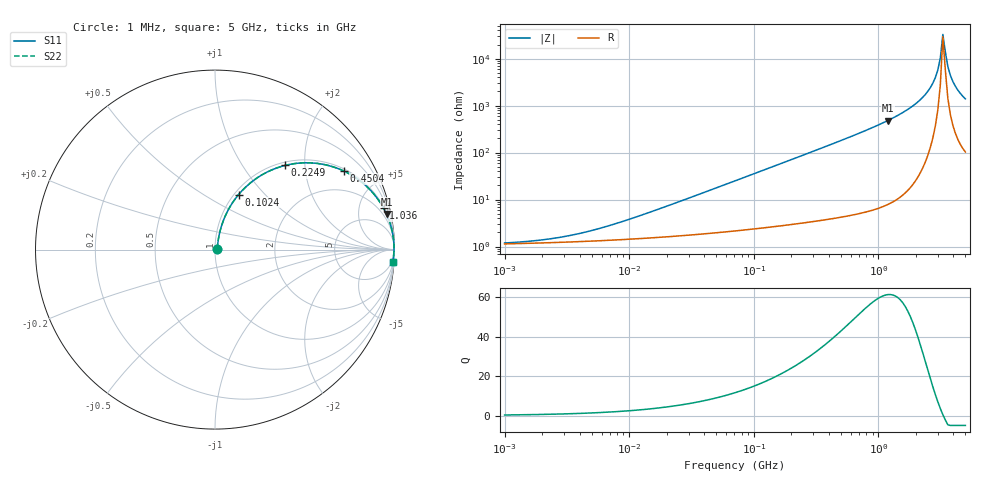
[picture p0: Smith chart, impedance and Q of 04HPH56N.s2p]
# MHz S MA R 50
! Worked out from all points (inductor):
!   185 points, 1 MHz to 5 GHz, reference 50 ohm
!   read as one part in series: L = 56 nH near 12.75 MHz
!   highest Q = 61.4 at 1.191 GHz (marker M1), where L = 64.3 nH
!   self-resonance near 3.296 GHz
!   S11 on the Smith chart (normalised r, x): 1 MHz: 1.02, +0.01; 102.4 MHz: 1.05, +0.72; 224.9 MHz: 1.06, +1.59; 450.4 MHz: 1.08, +3.23; 1.036 GHz: 1.13, +8.08; 5 GHz: 3, -28
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1  0.01176 17.0  0.9888 -0.2  0.9888 -0.2  0.01176 17.0
2.19661  0.01412 32.3  0.9881 -0.4  0.9881 -0.4  0.01412 32.3
4.19948  0.01929 48.3  0.9873 -0.8  0.9873 -0.8  0.01929 48.3
17.6357  0.06291 72.3  0.9827 -3.5  0.9827 -3.5  0.06291 72.3
70.7107  0.2376 71.4  0.9512 -13.7  0.9512 -13.7  0.2376 71.4
102.402  0.333 66.8  0.9213 -19.4  0.9213 -19.4  0.333 66.8
224.938  0.6113 50.1  0.7683 -37.7  0.7683 -37.7  0.6113 50.1
296.948  0.714 42.6  0.6776 -45.5  0.6776 -45.5  0.714 42.6
450.411  0.8409 31.4  0.5207 -57.2  0.5207 -57.2  0.8409 31.4
1036.25  0.967 13.8  0.2394 -75.2  0.2394 -75.2  0.967 13.8
1190.62  0.9759 11.7  0.203 -77.4  0.203 -77.4  0.9759 11.7
1247.03  0.9784 11.0  0.1915 -78.0  0.1915 -78.0  0.9784 11.0
1981.11  0.9937 5.3  0.09186 -83.4  0.09186 -83.4  0.9937 5.3
2615.33  0.997 2.4  0.04125 -84.6  0.04125 -84.6  0.997 2.4
2869.02  0.9973 1.4  0.02522 -83.2  0.02522 -83.2  0.9973 1.4
3004.94  0.9974 1.0  0.01734 -80.9  0.01734 -80.9  0.9974 1.0
3147.31  0.9974 0.5  0.009597 -73.8  0.009597 -73.8  0.9974 0.5
3296.42  0.9973 0.1  0.003047 -26.1  0.003047 -26.1  0.9973 0.1
3616.17  0.9968 -0.8  0.01478 77.1  0.01478 77.1  0.9968 -0.8
3787.49  0.9964 -1.3  0.02261 80.3  0.02261 80.3  0.9964 -1.3
4154.87  0.9954 -2.2  0.03854 82.1  0.03854 82.1  0.9954 -2.2
5000  0.9922 -4.1  0.0714 81.7  0.0714 81.7  0.9922 -4.1
